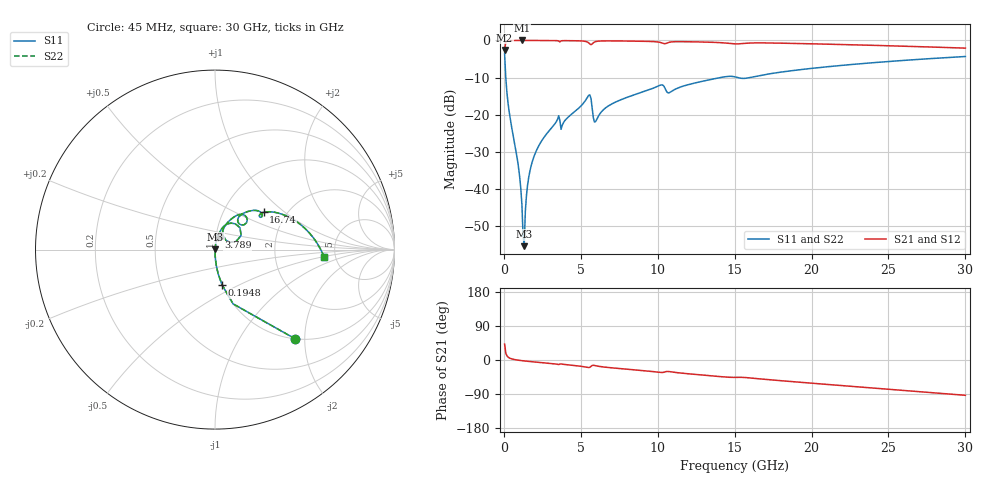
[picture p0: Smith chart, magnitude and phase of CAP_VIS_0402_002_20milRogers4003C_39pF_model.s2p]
! S-parameter model data by Modelithics Inc.  support@modelithics.com  813-866-6335  Tampa FL USA
! S-Parameter data specifications:
! Substrate: 20-mil Rogers 4003C, substrate thickness, H=0.508mm, Dielectric constant, Er=3.75
! PCB Mounting Pad Footprint: Pad width, PadW=0.50mm , Pad length, PadL=0.50mm , Pad gap, PadG (edge-to-edge)=0.40mm , Reference planes=1.4mm apart
! Created Wed Nov 18 12:54:40 2015
# hz S ma R 50
! 2 Port Network Data from SP1.SP block
! freq  magS11  angS11  magS21  angS21  magS12  angS12  magS22  angS22
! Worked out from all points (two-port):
!   401 points, 45 MHz to 30 GHz, reference 50 ohm
!   highest |S21| = -0.01 dB at 1.168 GHz (marker M1); lowest = -2.6 dB at 45 MHz (marker M2)
!   |S21| within 3 dB of the highest: start of sweep to end of sweep
!   lowest |S11| = -55.3 dB at 1.318 GHz (marker M3), VSWR 1.00, Z = 50.1 + j0.14 ohm
!   |S11| at or under -10 dB: 121.1 MHz to 14.05 GHz (13.93 GHz wide, 197 % of centre); 15.21 GHz to 15.97 GHz (761.7 MHz wide, 4.89 % of centre)
!   |S22| runs from -55.3 to -3.5 dB; largest |S21 - S12| = 0
!   S11 on the Smith chart (normalised r, x): 45 MHz: 1.00, -1.80; 194.8 MHz: 1.00, -0.41; 3.789 GHz: 1.03, +0.14; 16.74 GHz: 1.54, +0.72; 30 GHz: 4.04, -0.49
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4.5e7  0.6699 -48.0  0.7423 42.0  0.7423 42.0  0.6699 -48.0
1.94775e8  0.1998 -78.7  0.9794 11.2  0.9794 11.2  0.1998 -78.7
4.194375e8  0.08636 -85.4  0.9957 4.2  0.9957 4.2  0.08636 -85.4
9.4365e8  0.02004 -88.3  0.999 -0.6  0.999 -0.6  0.02004 -88.3
1.168312e9  0.006283 -83.7  0.9991 -1.8  0.9991 -1.8  0.006283 -83.7
1.318088e9  0.001714 54.4  0.999 -2.5  0.999 -2.5  0.001714 54.4
1.392975e9  0.005042 76.2  0.999 -2.8  0.999 -2.8  0.005042 76.2
1.692525e9  0.01762 82.5  0.9987 -4.1  0.9987 -4.1  0.01762 82.5
2.066962e9  0.03146 82.3  0.9983 -5.5  0.9983 -5.5  0.03146 82.3
3.414938e9  0.08147 76.7  0.9931 -10.8  0.9931 -10.8  0.08147 76.7
3.789375e9  0.07206 74.4  0.9915 -11.0  0.9915 -11.0  0.07206 74.4
5.062462e9  0.135 69.8  0.983 -16.9  0.983 -16.9  0.135 69.8
5.511788e9  0.1828 51.7  0.927 -19.9  0.927 -19.9  0.1828 51.7
5.961112e9  0.08123 51.6  0.9649 -15.0  0.9649 -15.0  0.08123 51.6
7.009538e9  0.1399 67.3  0.985 -20.7  0.985 -20.7  0.1399 67.3
1.007992e10  0.2465 52.7  0.9481 -32.4  0.9481 -32.4  0.2465 52.7
1.075391e10  0.1982 49.1  0.945 -30.6  0.945 -30.6  0.1982 49.1
1.50225e10  0.3238 35.7  0.8992 -45.8  0.8992 -45.8  0.3238 35.7
1.674491e10  0.3407 37.5  0.9262 -50.2  0.9262 -50.2  0.3407 37.5
2.003996e10  0.4216 27.9  0.9004 -61.3  0.9004 -61.3  0.4216 27.9
2.505742e10  0.5218 12.1  0.8472 -77.4  0.8472 -77.4  0.5218 12.1
3e10  0.6078 -3.6  0.7878 -93.2  0.7878 -93.2  0.6078 -3.6
